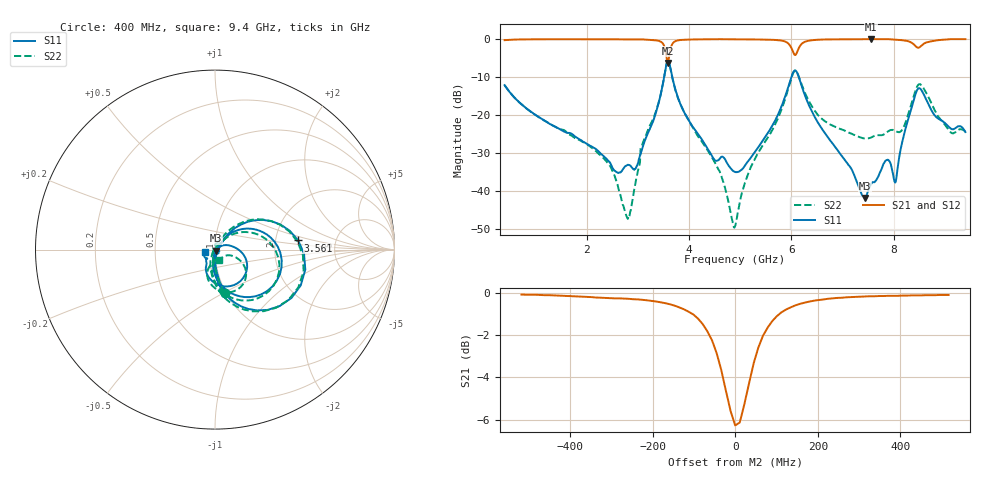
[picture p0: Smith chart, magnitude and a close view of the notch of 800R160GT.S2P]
!  American Technical Ceramics  Date:  6/19/09
!  One Norden Lane
!  Huntington Station,  NY.  11746-2102
!  Tel:  (631) 622-4700  Fax:  (631) 622-4748
!  Part Number  800R160GT
!  Description: Ultra-low ESR, NPO  Mounting Orientation: Horizontal
!  Application: High RF power Filters, Combiners, Matching networks,
!  Antenna, DC block, Bypass and Couplers
# GHZ S DB R 50
! Freq  |S11|  S11 Ph  |S21|  S21 Ph  |S12|  S12 Ph  |S22|  S22 Ph
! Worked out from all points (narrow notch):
!   801 points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, 400 MHz to 9.4 GHz, reference 50 ohm
!   highest |S21| = 0.00 dB at 7.555 GHz (marker M1); lowest = -6.3 dB at 3.584 GHz (marker M2)
!   notch at M2: 6.2 dB deep, 87.5 MHz wide at half that depth
!   lowest |S11| = -41.8 dB at 7.431 GHz (marker M3), VSWR 1.02, Z = 50.5 - j0.666 ohm
!   |S11| at or under -10 dB: start of sweep to 3.515 GHz; 3.676 GHz to 6.001 GHz (2.326 GHz wide, 48.1 % of centre); 6.146 GHz to end of sweep
!   |S22| runs from -49.7 to -5.8 dB; largest |S21 - S12| = 0.0013
!   S11 on the Smith chart (normalised r, x): 400 MHz: 0.99, -0.51; 3.561 GHz: 2.69, +0.35; 9.4 GHz: 0.89, -0.03
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0.4  -12.13 -77.3  -0.28 12.4  -0.28 12.4  -12.14 -77.6
1.908  -26.76 -87.9  -0.03 -6.2  -0.03 -6.2  -26.93 -102.9
2.448  -32.35 -73.2  -0.04 -9.9  -0.04 -9.9  -33.20 -121.5
2.808  -33.10 -18.3  -0.10 -12.4  -0.11 -12.4  -47.34 -136.5
2.976  -33.66 17.8  -0.06 -13.8  -0.06 -13.8  -36.32 130.5
3.404  -17.09 48.6  -0.45 -22.2  -0.45 -22.3  -16.92 52.8
3.561  -6.63 6.3  -4.59 -31.6  -4.59 -31.6  -6.71 5.6
3.584  -5.76 -12.5  -6.27 -17.4  -6.27 -17.4  -5.87 -14.0
3.786  -15.44 -85.9  -0.34 -6.3  -0.34 -6.3  -15.55 -93.0
4.585  -31.79 -48.7  -0.03 -17.4  -0.03 -17.4  -34.50 -129.2
4.9  -34.99 -21.9  -0.07 -19.9  -0.07 -19.9  -49.34 138.6
5.181  -31.71 25.7  -0.09 -22.0  -0.09 -22.0  -34.64 65.5
5.598  -23.52 47.3  -0.18 -26.0  -0.18 -26.0  -24.70 49.3
6.048  -8.51 -8.4  -3.81 -31.9  -3.81 -31.9  -8.67 -13.1
6.408  -19.23 -94.7  -0.29 -19.1  -0.29 -19.1  -17.84 -97.1
7.431  -41.82 -54.4  -0.03 -29.1  -0.03 -29.0  -26.17 -78.7
7.555  -38.23 -27.4  0.00 -30.0  0.00 -30.0  -25.96 -69.8
7.904  -31.98 -27.6  -0.03 -33.5  -0.03 -33.4  -24.21 -54.8
8.039  -37.62 5.9  -0.16 -35.0  -0.16 -35.0  -24.18 -53.9
8.489  -12.94 -50.7  -2.26 -32.1  -2.26 -32.1  -11.92 -56.5
9.096  -23.35 -132.5  -0.03 -31.7  -0.03 -31.7  -24.31 -92.6
9.4  -24.48 -165.2  -0.01 -35.3  -0.01 -35.3  -24.35 -68.6
